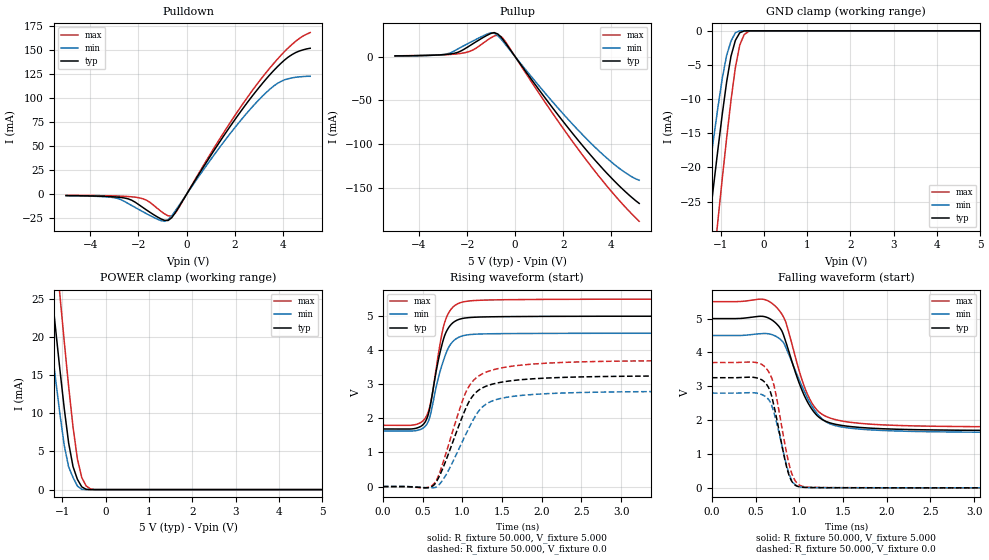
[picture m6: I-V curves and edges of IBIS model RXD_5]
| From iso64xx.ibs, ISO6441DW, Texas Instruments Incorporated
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|   RXD_5 Model
[Model]   RXD_5
Model_type   3-state
Vmeas = 2.2V   |Reference voltage for timing measurements
Cref = 15pF   |Timing specification test load capacitance value
Vref = 0   |Timing specification test load voltage; GND
| variable   typ   min   max
C_comp   2.1pF   1.7pF   2.5pF
|   typ   min   max
[Temperature Range]   25.0   -40   125
[Voltage range]   5.0V   4.5V   5.5V
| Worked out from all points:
|   slope of the pulldown table from 0 to 0.75 V, typ, clamps not added: 24.7 ohm
|   slope of the pullup table from 0 to 0.75 V, typ, clamps not added: 26.2 ohm
|   GND clamp passes 1 mA (typ) near -0.62 V on its own axis
|   POWER clamp passes 1 mA (typ) near -0.62 V on its own axis
|   rising waveform, R_fixture 50.000, V_fixture 5.000: 20-80 % time 170ps typ, 189ps min, 162ps max; typ from 1.69 V to 5 V
|   rising waveform, R_fixture 50.000, V_fixture 0.0: 20-80 % time 340ps typ, 370ps min, 327ps max; typ from 0 V to 3.25 V
|   falling waveform, R_fixture 50.000, V_fixture 5.000: 20-80 % time 294ps typ, 318ps min, 276ps max; typ from 5 V to 1.69 V
|   falling waveform, R_fixture 50.000, V_fixture 0.0: 20-80 % time 158ps typ, 157ps min, 163ps max; typ from 3.25 V to 0 V
[Pulldown]
|Voltage   I(typ)   I(min)   I(max)
-5V       -1.578mA   -1.684mA   -1.347mA
-3.037V   -2.834mA   -3.646mA   -1.883mA
-2.433V   -4.915mA   -9.695mA   -2.538mA
-1.98V    -11.08mA   -16.09mA   -3.834mA
-923mV    -27.28mA   -28.28mA   -20.47mA
-621mV    -24.59mA   -22.76mA   -22.99mA
-319mV    -13.14mA   -11.79mA   -13.88mA
1.493V    58.93mA    52.74mA    62.23mA
3.154V    115.4mA    102.1mA    121.9mA
3.758V    132.2mA    114.9mA    140mA
4.211V    142.3mA    119.8mA    151.9mA
5.117V    151.4mA    122.3mA    167.7mA
[Pullup]
|Voltage   I(typ)   I(min)   I(max)
-5V       836.1uA    694.4uA    925.8uA
-2.986V   2.249mA    2.428mA    2.059mA
-2.231V   6.782mA    11.08mA    3.8mA
-1.778V   14.36mA    17.55mA    7.299mA
-1.023V   26.29mA    27.16mA    21.23mA
-872mV    27.46mA    26.96mA    23.52mA
-721mV    25.84mA    23.78mA    24.65mA
-570mV    21.75mA    19.62mA    22.79mA
1.393V    -52.39mA   -46.24mA   -57.94mA
2.903V    -104.6mA   -91.78mA   -115.8mA
4.262V    -145.5mA   -125.9mA   -161.8mA
5.168V    -167.5mA   -141.1mA   -187.9mA
[GND_clamp]
|Voltage   I(typ)   I(min)   I(max)
-5V       -243.7mA   -207.1mA   -289.1mA
-1.465V   -39.55mA   -30.35mA   -53.49mA
-1.364V   -33.9mA    -25.46mA   -46.98mA
-1.263V   -28.3mA    -20.61mA   -40.51mA
-1.061V   -17.39mA   -11.24mA   -27.81mA
-859mV    -7.484mA   -3.592mA   -15.71mA
-758mV    -3.707mA   -1.499mA   -10.16mA
-657mV    -1.398mA   -276.8uA   -5.372mA
-556mV    -278.8uA   -7.348uA   -2.077mA
-455mV    -16.52uA   -48.33nA   -563.2uA
-354mV    -408.3nA   -367.3pA   -87.25uA
5V        0A         0A         0A
[POWER_clamp]
|Voltage   I(typ)   I(min)   I(max)
-5V       245mA      208mA      291.3mA
-1.464V   38.03mA    29.15mA    51.43mA
-1.363V   32.33mA    24.21mA    44.83mA
-1.262V   26.69mA    19.32mA    38.3mA
-1.06V    15.74mA    9.932mA    25.51mA
-959mV    10.61mA    5.771mA    19.37mA
-858mV    6.112mA    2.974mA    13.52mA
-757mV    3.021mA    1.593mA    8.217mA
-656mV    1.346mA    467.6uA    4.021mA
-555mV    361.6uA    25.6uA     1.575mA
-252mV    28.8nA     42.83pA    9.374uA
5V        0A         0A         0A
[Ramp]
| variable   typ   min   max
dV/dt_r   1.952/0.340n   1.679/0.370n   2.221/0.327n
dV/dt_f   1.986/0.294n   1.720/0.318n   2.221/0.276n
R_load = 50.000
[Rising Waveform]
R_fixture= 50.000
V_fixture= 5.000
V_fixture_min= 4.500
V_fixture_max= 5.500
|time   V(typ)   V(min)   V(max)
0s        1.69V      1.633V     1.798V
393ps     1.699V     1.635V     1.809V
528ps     1.879V     1.757V     1.988V
602ps     2.441V     2.138V     2.463V
699ps     3.718V     3.19V      3.892V
746ps     4.18V      3.576V     4.511V
789ps     4.492V     3.872V     4.892V
907ps     4.849V     4.311V     5.315V
1.094ns   4.961V     4.46V      5.449V
15ns      5V         4.5V       5.5V
[Rising Waveform]
R_fixture= 50.000
V_fixture= 0.0
V_fixture_min= 0.0
V_fixture_max= 0.0
|time   V(typ)   V(min)   V(max)
0s        706.9nV    257.4nV    1.82uV
623ps     10.62mV    -37.24mV   39.48mV
690ps     210.3mV    16.95mV    259.7mV
779ps     677.1mV    281.1mV    860.1mV
1.01ns    2.107V     1.367V     2.568V
1.1ns     2.553V     1.795V     2.998V
1.211ns   2.836V     2.228V     3.252V
1.33ns    2.972V     2.462V     3.384V
1.76ns    3.14V      2.678V     3.569V
15ns      3.253V     2.799V     3.701V
[Falling Waveform]
R_fixture= 50.000
V_fixture= 5.000
V_fixture_min= 4.500
V_fixture_max= 5.500
|time   V(typ)   V(min)   V(max)
0s        5V         4.5V       5.5V
575ps     5.067V     4.556V     5.574V
701ps     4.932V     4.513V     5.424V
790ps     4.682V     4.372V     5.172V
838ps     4.376V     4.192V     4.944V
1.036ns   2.851V     2.972V     3.149V
1.166ns   2.246V     2.327V     2.418V
1.356ns   1.915V     1.886V     2.059V
1.694ns   1.784V     1.734V     1.906V
15ns      1.69V      1.633V     1.798V
[Falling Waveform]
R_fixture= 50.000
V_fixture= 0.0
V_fixture_min= 0.0
V_fixture_max= 0.0
|time   V(typ)   V(min)   V(max)
0s        3.253V     2.799V     3.701V
482ps     3.263V     2.808V     3.711V
633ps     3.029V     2.655V     3.493V
672ps     2.814V     2.513V     3.319V
718ps     2.331V     2.148V     2.945V
840ps     780.7mV    818.2mV    1.226V
895ps     293.5mV    328.6mV    583.6mV
975ps     50.57mV    57.23mV    138.9mV
1.093ns   11.51mV    9.535mV    22mV
15ns      1.18nV     757.4pV    141.3nV
